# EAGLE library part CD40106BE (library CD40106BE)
CD40106BE, CMOS Hex Schmitt Inverter, 4.2mA 3 18 V 14-Pin PDIP Source: Datasheet
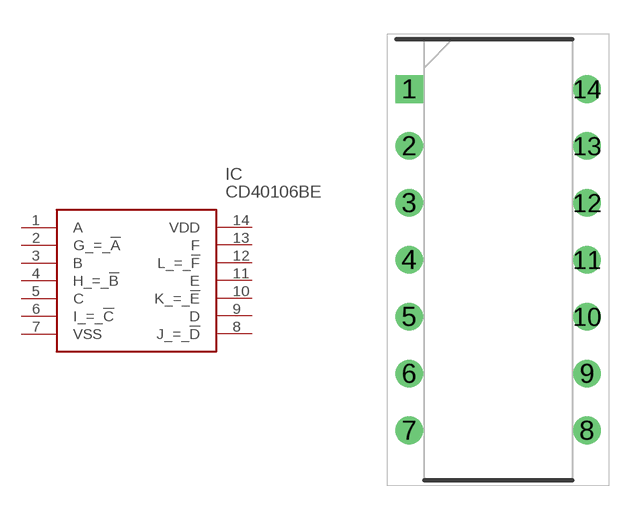
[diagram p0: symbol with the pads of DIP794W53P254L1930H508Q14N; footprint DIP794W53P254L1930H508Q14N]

Designator prefix IC

## CD40106BE (Arrow_Part_Number: CD40106BE; Arrow_Price-Stock: https://www.arrow.com/en/products/cd40106be/texas-instruments?region=nac; Description: CD40106BE, CMOS Hex Schmitt Inverter, 4.2mA 3 18 V 14-Pin PDIP; Height: 5.08mm; Manufacturer_Name: Texas Instruments; Manufacturer_Part_Number: CD40106BE; Mouser_Part_Number: 595-CD40106BE; Mouser_Price-Stock: https://www.mouser.co.uk/ProductDetail/Texas-Instruments/CD40106BE?qs=YhsVCygOPE1CyKyInx%252Bh3Q%3D%3D)  [DIP794W53P254L1930H508Q14N]
1  A
2  G_=_!A
3  B
4  H_=_!B
5  C
6  I_=_!C
7  VSS
8  J_=_!D
9  D
10  K_=_!E
11  E
12  L_=_!F
13  F
14  VDD

## Footprint DIP794W53P254L1930H508Q14N (pad centres in mm)
N (R-PDIP-T)
drill 0.73 pad 1.13 square: 1 -3.97,7.62
drill 0.73 pad 1.13: 2 -3.97,5.08; 3 -3.97,2.54; 4 -3.97,0; 5 -3.97,-2.54; 6 -3.97,-5.08; 7 -3.97,-7.62; 8 3.97,-7.62; 9 3.97,-5.08; 10 3.97,-2.54; 11 3.97,0; 12 3.97,2.54; 13 3.97,5.08; 14 3.97,7.62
